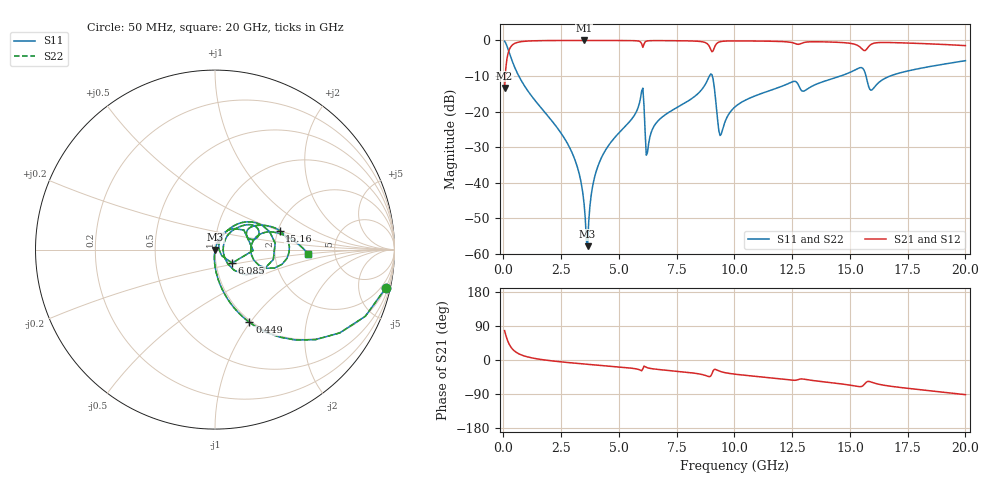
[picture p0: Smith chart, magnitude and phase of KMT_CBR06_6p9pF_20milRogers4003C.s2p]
! Data measured by Modelithics Inc. support@modelithics.com 813-866-6335
! KEMET CBR0603 6.9pF, Pad Width= 0.851mm, Pad Length= 0.64mm, Pad Gap= 0.62mm, 20mil Rogers 4003C substrate Data, January 2022
# hz S ma R 50
! 2 Port Network Data from SP1.SP block
! freq  magS11  angS11  magS21  angS21  magS12  angS12  magS22  angS22
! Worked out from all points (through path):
!   401 points, 50 MHz to 20 GHz, reference 50 ohm
!   highest |S21| = -0.01 dB at 3.491 GHz (marker M1); lowest = -13.4 dB at 50 MHz (marker M2)
!   group delay of S21, straight-line fit = 14 ps
!   lowest |S11| = -57.9 dB at 3.641 GHz (marker M3), VSWR 1.00, Z = 50.1 + j0.0529 ohm
!   |S11| at or under -10 dB: 663.8 MHz to 8.919 GHz (8.255 GHz wide, 172 % of centre); 9.042 GHz to 14.6 GHz (5.557 GHz wide, 47 % of centre); 15.7 GHz to 16.75 GHz (1.054 GHz wide, 6.5 % of centre)
!   |S22| runs from -57.9 to -0.2 dB; largest |S21 - S12| = 0
!   S11 on the Smith chart (normalised r, x): 50 MHz: 0.98, -9.03; 449 MHz: 0.98, -0.99; 6.085 GHz: 1.20, -0.18; 15.16 GHz: 2.04, +0.50; 20 GHz: 3.14, -0.19
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5e7  0.9768 -12.5  0.2138 77.5  0.2138 77.5  0.9768 -12.5
2.495e8  0.6735 -48.4  0.7387 41.6  0.7387 41.6  0.6735 -48.4
4.49e8  0.4481 -64.7  0.8934 25.2  0.8934 25.2  0.4481 -64.7
2.793125e9  0.03445 -95.2  0.9984 -6.7  0.9984 -6.7  0.03445 -95.2
3.391625e9  0.008846 -93.6  0.9988 -10.0  0.9988 -10.0  0.008846 -93.6
3.491375e9  0.005019 -88.9  0.9989 -10.6  0.9989 -10.6  0.005019 -88.9
3.641e9  0.001275 24.4  0.9988 -11.3  0.9988 -11.3  0.001275 24.4
3.890375e9  0.009935 71.1  0.9987 -12.6  0.9987 -12.6  0.009935 71.1
4.289375e9  0.02406 72.5  0.9984 -14.7  0.9984 -14.7  0.02406 72.5
5.93525e9  0.1551 49.2  0.9514 -27.0  0.9514 -27.0  0.1551 49.2
6.084875e9  0.1214 -38.0  0.8861 -16.2  0.8861 -16.2  0.1214 -38.0
6.2345e9  0.02633 35.6  0.9848 -20.5  0.9848 -20.5  0.02633 35.6
6.73325e9  0.07623 62.6  0.9938 -25.2  0.9938 -25.2  0.07623 62.6
8.977625e9  0.3371 6.0  0.7429 -42.2  0.7429 -42.2  0.3371 6.0
9.376625e9  0.04595 -4.5  0.958 -30.0  0.958 -30.0  0.04595 -4.5
1.0025e10  0.1161 48.5  0.9847 -37.4  0.9847 -37.4  0.1161 48.5
1.336662e10  0.2277 32.1  0.9577 -53.9  0.9577 -53.9  0.2277 32.1
1.516212e10  0.3752 16.5  0.8909 -68.0  0.8909 -68.0  0.3752 16.5
1.556112e10  0.4043 -6.9  0.7393 -68.0  0.7393 -68.0  0.4043 -6.9
1.591025e10  0.1993 -0.8  0.8771 -57.9  0.8771 -57.9  0.1993 -0.8
1.670825e10  0.3124 18.4  0.934 -68.8  0.934 -68.8  0.3124 18.4
2e10  0.5187 -2.5  0.8448 -91.4  0.8448 -91.4  0.5187 -2.5
